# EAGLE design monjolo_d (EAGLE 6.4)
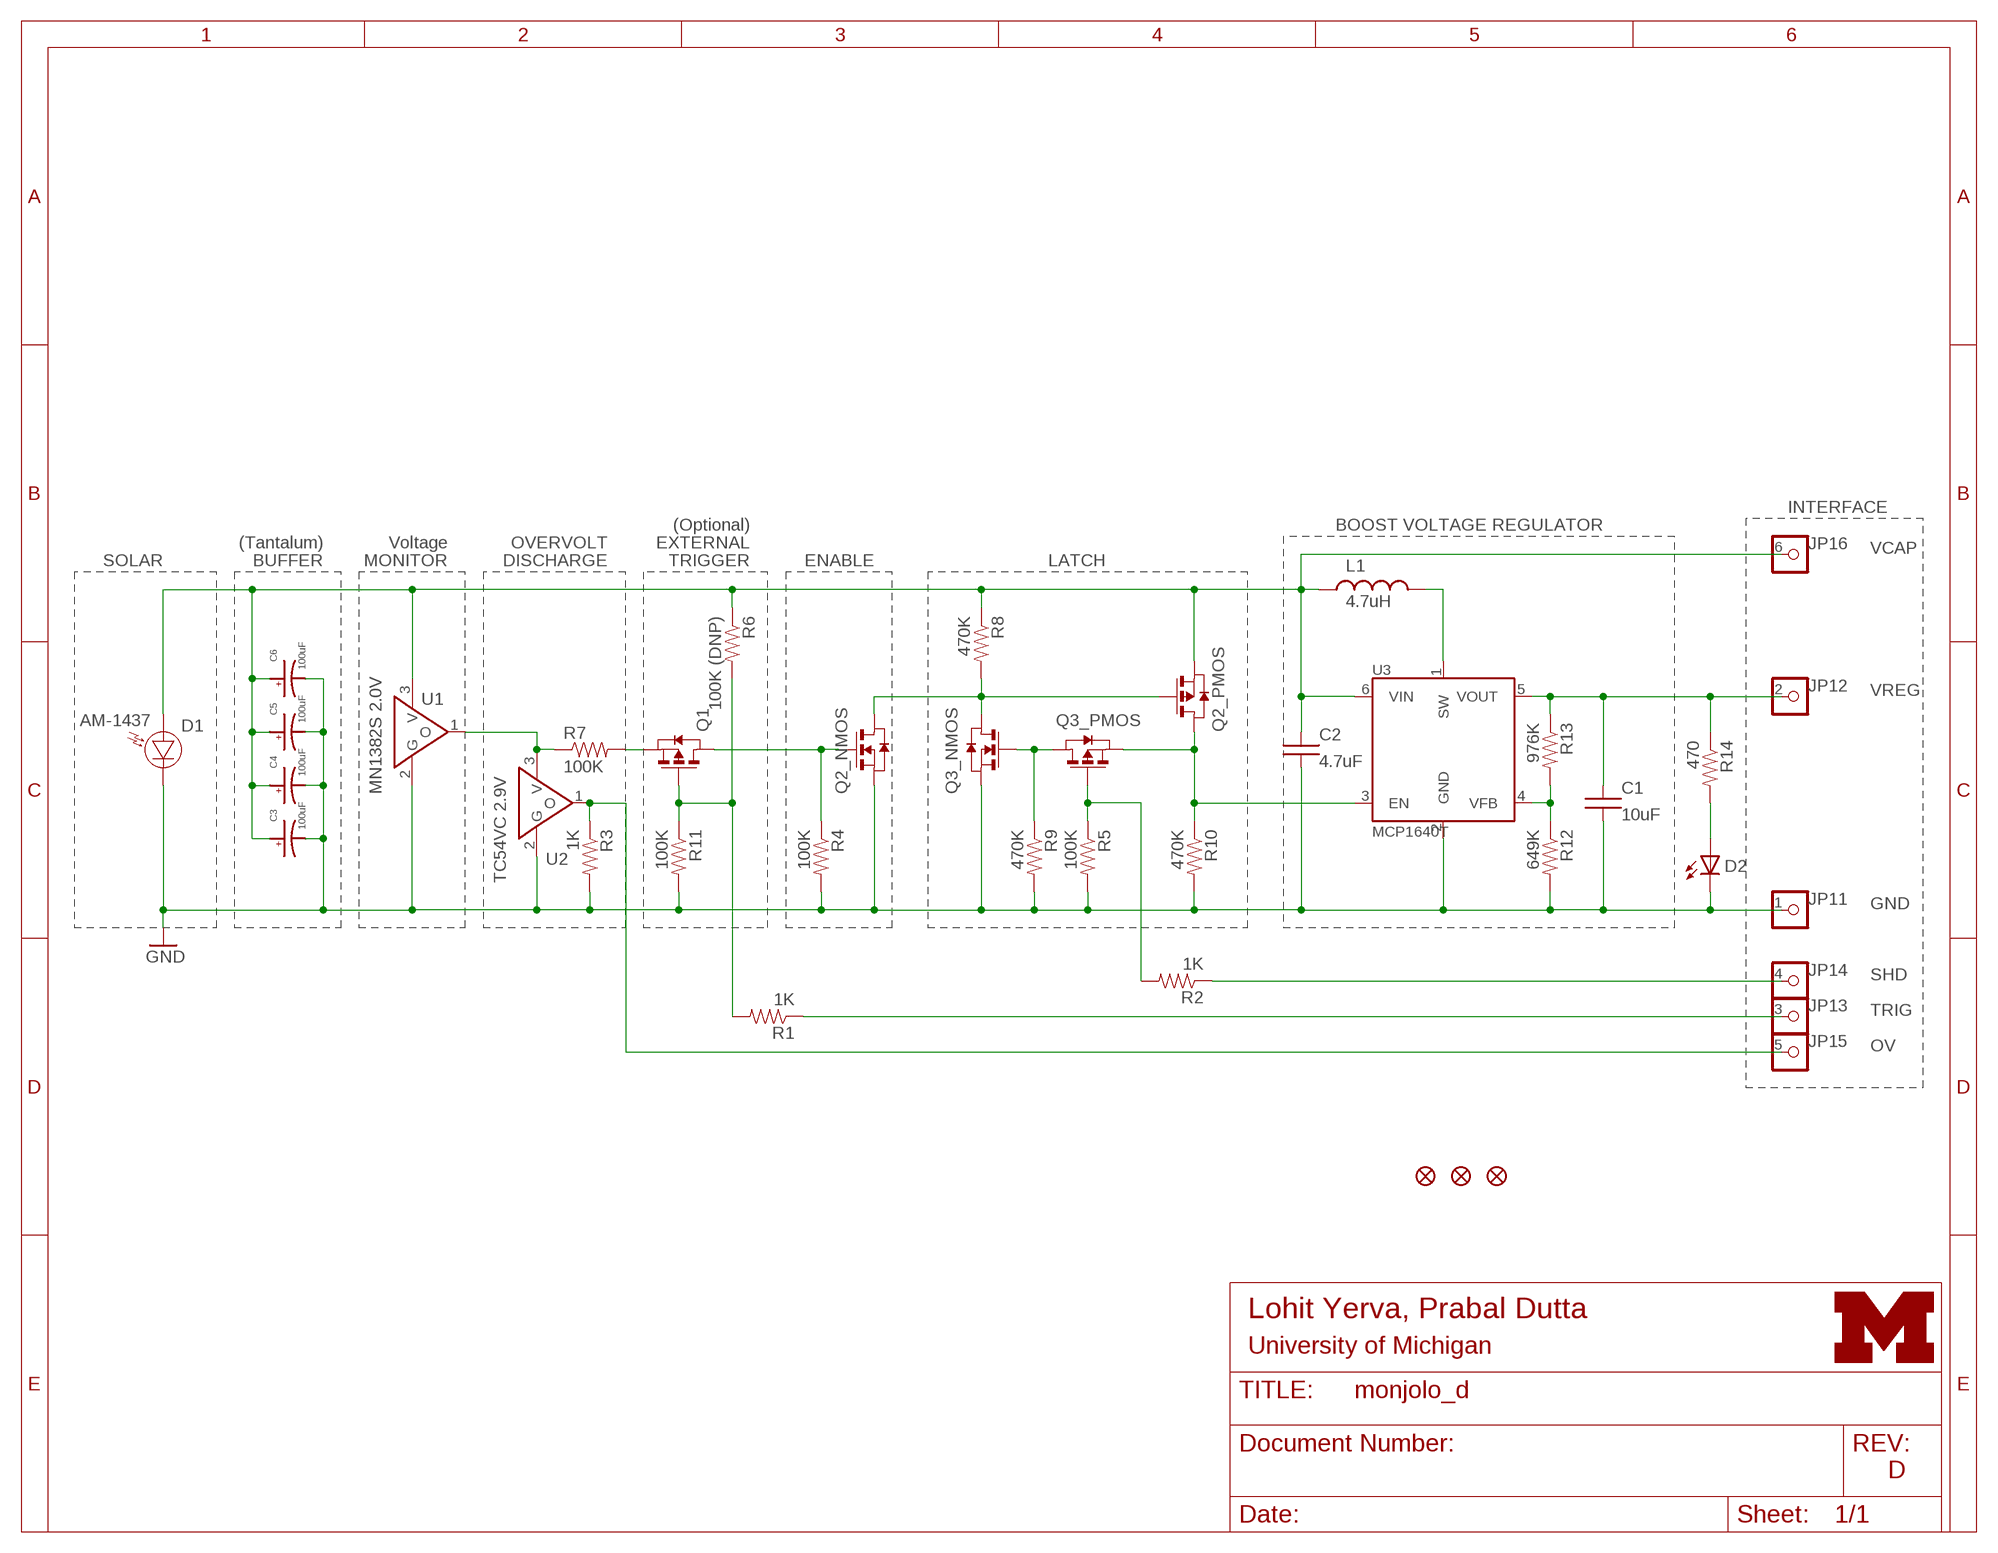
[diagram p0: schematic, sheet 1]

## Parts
C1  10uF  CAP  [R0603B]
C2  4.7uF  CAP  [R0603B]
C3  100uF  1210_CAP_POLARIZED  [CAP1210]
C4  100uF  1210_CAP_POLARIZED  [CAP1210]
C5  100uF  1210_CAP_POLARIZED  [CAP1210]
C6  100uF  1210_CAP_POLARIZED  [CAP1210]
D1  AM-1437  [AM-1437]
D2  LED0603  [LED-0603]
JP1  PINHD6  [HD6]
JP2  FIDUCIAL1X2  [FIDUCIAL-1X2]
JP3  FIDUCIAL1X2  [FIDUCIAL-1X2]
JP4  FIDUCIAL1X2  [FIDUCIAL-1X2]
L1  4.7uH  L-US  [L2828]
Q1  PMOSSOT23  [SOT-23]
Q2  DUAL_MOSFET_NP  [TSOP-6]
Q3  DUAL_MOSFET_NP  [TSOP-6]
R1  1K  RESISTOR  [R0603B]
R2  1K  RESISTOR  [R0603B]
R3  1K  RESISTOR  [R0603B]
R4  100K  RESISTOR  [R0603B]
R5  100K  RESISTOR  [R0603B]
R6  100K (DNP)  RESISTOR  [R0603B]
R7  100K  RESISTOR  [R0603B]
R8  470K  RESISTOR  [R0603B]
R9  470K  RESISTOR  [R0603B]
R10  470K  RESISTOR  [R0603B]
R11  100K  RESISTOR  [R0603B]
R12  649K  RESISTOR  [R0603B]
R13  976K  RESISTOR  [R0603B]
R14  470  RESISTOR  [R0603B]
U1  MN1382S 2.0V  MN1382S  [MINI-3DC]
U2  TC54VC 2.9V  MN1382S  [MINI-3DC]
U3  MCP1640T  MCP1640  [SOT-23-6]
U$1  UMICH_SOLID_SMALL  [UMICH_SOLID_75MIL]

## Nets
GND: C1.2 C2.2 C3.ANODE C4.ANODE C5.ANODE C6.ANODE D1.-(C) D2.C JP1.1 Q2.5(_NMOS:S) Q3.5(_NMOS:S) R3.2 R4.2 R5.2 R9.2 R10.2 R11.2 R12.2 U1.2(G) U2.2(G) U3.2(GND)
N$1: R12.1 R13.2 U3.4(VFB)
N$2: Q1.2(S) R7.2
N$3: JP1.3 R1.1
N$4: L1.2 U3.1(SW)
N$5: D2.A R14.2
N$6: Q3.1(_NMOS:G) Q3.4(_PMOS:D) R9.1
N$7: Q1.1(D) Q2.1(_NMOS:G) R4.1
N$8: JP1.4 R2.1
N$9: Q2.3(_PMOS:G) Q2.6(_NMOS:D) Q3.6(_NMOS:D) R8.2
N$12: Q3.3(_PMOS:G) R2.2 R5.1
N$13: JP1.5 R3.1 U2.1(O)
N$14: R7.1 U1.1(O) U2.3(V)
N$15: Q1.3(G) R1.2 R6.2 R11.1
N$18: Q2.4(_PMOS:D) Q3.2(_PMOS:S) R10.1 U3.3(EN)
VCAP: C2.1 C3.CATHODE C4.CATHODE C5.CATHODE C6.CATHODE D1.+(A) JP1.6 L1.1 Q2.2(_PMOS:S) R6.1 R8.1 U1.3(V) U3.6(VIN)
VREG: C1.1 JP1.2 R13.1 R14.1 U3.5(VOUT)

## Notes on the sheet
- INTERFACE
- (Optional) | BOOST VOLTAGE REGULATOR
- (Tantalum) | Voltage | OVERVOLT | EXTERNAL
- SOLAR | BUFFER | MONITOR | DISCHARGE | TRIGGER | ENABLE | LATCH | VCAP
- VREG
- GND
- SHD
- TRIG
- OV
- Lohit Yerva, Prabal Dutta
- University of Michigan
- D

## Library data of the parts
C1 C2 = Gecko:CAP
C3-C6 = Gecko:1210_CAP_POLARIZED
D1 = umich:AM-1437
D2 = umich:LED: LEDs
JP1 = Gecko:PINHD6
JP2-JP4 = SparkFun-Aesthetics:FIDUCIAL: Fiducial Alignment Points
L1 = Gecko:L-US
Q1 = berkeley-epic:PMOSSOT23: MOS FET
Q2 Q3 =  gecko_vreg_revC:DUAL_MOSFET_NP
R1-R14 = Gecko:RESISTOR
U1 U2 = umich:MN1382S
U3 = Gecko:MCP1640
U$1 = logos:UMICH_SOLID

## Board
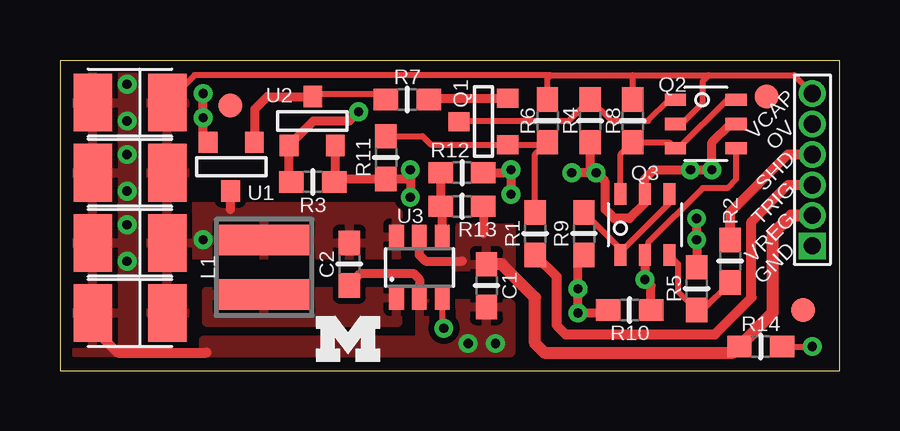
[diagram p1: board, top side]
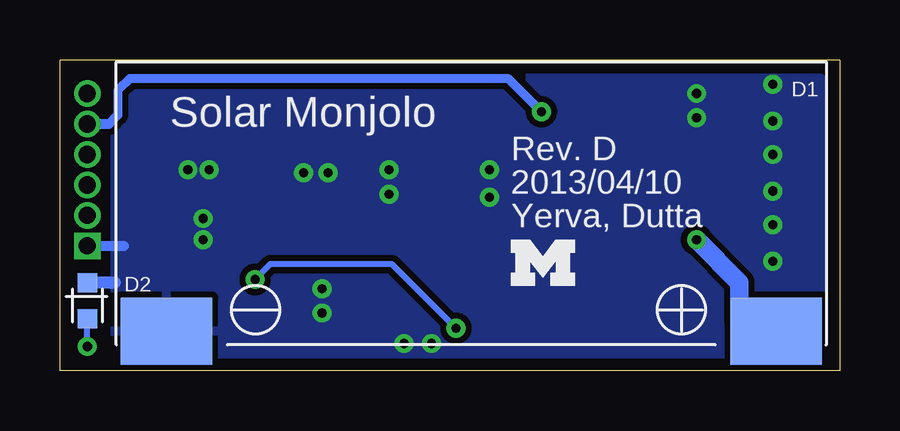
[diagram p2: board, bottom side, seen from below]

Size 32.51 x 12.95 mm. Coordinates in mm from the lower left corner, seen from the top.
Outline: 32.51,0 32.51,12.95 0,12.95 0,0 32.51,0
Copper layers (1*16): Top 0.0178mm / dielectric 59mil / Bottom 0.0178mm
Design rules "SSC-EAGLE-2Lyr_v1.0.0.3 *": minimum track width 6mil, minimum drill 14mil, track to track 6mil, track to pad 6mil, pad to pad 6mil, via to via 6mil, smd to smd 6mil, copper to edge 20mil, drill to drill 16mil, minimum pad ring 8mil, minimum via ring 8mil, stop-mask expansion 3mil, vias tented up to drill 20mil, thermal gap 10mil

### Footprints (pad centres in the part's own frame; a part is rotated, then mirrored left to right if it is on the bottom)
R0603B = smd 1.016 x 0.889: 1 -0.889,0; 2 0.889,0
CAP1210 = smd 2.4 x 1.6: ANODE 0,-1.55; CATHODE 0,1.55
AM-1437 = smd 3.81 x 2.794: + 12.7,-5.334; - -12.7,-5.334
LED-0603 = smd 0.8 x 0.8: A 0,-0.75; C 0,0.75
HD6 = drill 0.711 pad 1.016 square: 1 -2.54,0 | drill 0.711 pad 1.016: 2 -1.27,0; 3 0,0; 4 1.27,0; 5 2.54,0; 6 3.81,0
FIDUCIAL-1X2 = smd 1 x 1: 1 0,0
L2828 = smd 1.27 x 3.81: 1 -1.143,0; 2 1.143,0
SOT-23 = smd 0.787 x 0.889: 1 0.025,-1.016; 2 -0.94,1.016; 3 0.991,1.016
TSOP-6 = smd 0.508 x 0.889: 1 -1.016,-1.27; 2 0,-1.27; 3 1.016,-1.27; 4 1.016,1.27; 5 0,1.27; 6 -1.016,1.27
MINI-3DC = smd 0.787 x 0.889: 1 -0.991,-1.016; 2 0.94,-1.016; 3 0,1.016
SOT-23-6 = smd 0.61 x 1.016: 1 -0.953,-1.27; 2 0,-1.27; 3 0.953,-1.27; 4 0.953,1.27; 5 0,1.27; 6 -0.953,1.27

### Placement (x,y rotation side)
C1  17.78,3.56 270 top
C2  12.06,4.45 270 top
C3  2.92,11.18 270 top
C4  2.92,8.26 270 top
C5  2.92,5.33 270 top
C6  2.92,2.41 270 top
D1  15.37,6.99 0 bottom
D2  31.37,2.92 0 bottom
JP1  31.37,7.75 90 top
JP2  30.99,2.54 0 top
JP3  7.11,11.05 0 top
JP4  29.46,11.43 0 top
L1  8.51,4.32 270 top
Q1  17.65,10.41 270 top
Q2  26.92,10.29 270 top
Q3  24.38,6.1 0 top
R1  19.81,5.71 90 top
R2  27.94,4.57 270 top
R3  10.54,7.87 0 top
R4  22.1,10.41 270 top
R5  26.54,3.43 90 top
R6  20.32,10.41 270 top
R7  14.48,11.3 0 top
R8  23.88,10.41 270 top
R9  21.84,5.71 270 top
R10  23.75,2.54 180 top
R11  13.59,8.89 270 top
R12  16.76,8.26 0 top
R13  16.76,6.86 180 top
R14  29.21,1.02 0 top
U1  7.11,8.51 180 top
U2  10.54,10.41 0 top
U3  14.99,4.32 0 top
U$1  10.67,0.38 0 top
U$3  UMICH_SOLID_SMALL  [UMICH_SOLID_75MIL]  13.72,3.56 0 bottom

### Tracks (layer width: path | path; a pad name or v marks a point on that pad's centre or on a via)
GND  (via drill 0.38)
  Top 0.381: C2.2 12.09,3.62 12.53,4.06 14.73,4.06 14.99,3.81 U3.2 | U1.2 5.97,9.73 v5.97,10.54 v5.97,11.56 | R12.2 18.67,8.26 v18.8,8.38 v18.8,7.37 | v22.35,8.26 v21.34,8.26 | R10.2 23.11,2.41 v21.59,2.41 v21.59,3.43 21.59,4.57 R9.2 | v14.61,8.38 v14.61,7.24 14.61,8 R11.2 11.56,8 11.48,7.92 | R3.2 11.48,7.92 | 11.48,7.92 U2.2 | v26.54,6.35 v26.54,5.46 R5.2 | Q2.5 27.94,10.29 27.18,9.53 v27.18,8.38 v26.29,8.38 24.77,8.38 24.38,8 Q3.5 24.38,6.99 23.75,6.35 23.11,6.35 22.73,6.73 22.73,7.87 v22.35,8.26 | R4.2 22.1,8.51 v22.35,8.26
  Top 0.406: C6.ANODE 1.37,1.8 2.41,0.76 6.1,0.76
  Bottom 0.406: JP1.1 29.84,5.21
  Bottom 0.508: D2.C 30.36,3.67 30.23,3.68
  other vias: 18.16,1.14 17.02,1.14 2.79,4.57 2.79,6.1 2.79,7.49 2.79,9.02 2.79,10.41 2.79,11.94
  pour Bottom (isolate 0.254): 0.76,0.64 0.76,12.19 30.23,12.19 30.23,0.64
  pour Top (isolate 0.254): 5.97,1.27 5.97,0.76 18.8,0.76 18.8,2.79 14.99,2.79 14.99,1.27
  pour Top (isolate 0.305): 0.64,12.32 3.05,12.32 3.05,0.76 0.64,0.76
N$1
  Top 0.381: R12.1 R13.2 15.94,7.11 U3.4
N$2
  Top 0.381: R7.2 15.42,11.35 Q1.2
N$3
  Top 0.406: R1.1 20.7,3.94 20.7,1.91 21.08,1.52 27.3,1.52 28.83,3.05 28.83,6.22 30.35,7.75 JP1.3
N$4
  pour Top (isolate 0.254): 14.1,3.3 6.1,3.3 6.1,2.03 14.1,2.03
N$5  (via drill 0.38)
  Top 0.254: R14.2 v31.37,1.02
  Bottom 0.254: v31.37,1.02 D2.A
N$6
  Top 0.254: Q3.4 25.4,6.99 23.37,4.95 Q3.1 23.37,5.08 R9.1
N$7
  Top 0.254: Q1.1 16.66,10.41 21.21,10.41 R4.1 22.99,10.41 24.51,10.41 25.4,11.3 Q2.1
N$8
  Top 0.406: R2.1 27.94,6.6 30.35,9.02 JP1.4
N$9
  Top 0.254: Q2.6 27.81,11.3 25.78,9.27 Q2.3 25.4,9.53 R8.2 23.37,9.02 Q3.6
N$12
  Top 0.254: R2.2 26.8,2.54 R5.1 25.78,3.3 25.78,4.45 Q3.3
N$13  (via drill 0.38)
  Top 0.381: R3.1 9.55,7.98 U2.1 10.57,10.41 12.06,10.41 v12.45,10.79
  Bottom 0.381: 30.48,10.29 30.1,10.67 30.1,11.68 29.59,12.19 13.84,12.19 v12.45,10.79
  Bottom 0.406: 30.48,10.29 JP1.5
N$14
  Top 0.254: R7.1 13.34,11.56 10.79,11.56 U2.3
  Top 0.381: U2.3 8.64,11.43 8.13,10.92 8.13,9.93 U1.1
N$15
  Top 0.254: R11.1 15.11,9.78 15.47,9.42 Q1.3 20.34,9.42 R6.2 19.81,9.02 R1.2
N$18  (via drill 0.38)
  Top 0.254: U3.3 15.94,1.84 v16,1.78 | Q2.4 28.19,8 27.81,7.62 26.8,7.62 24.51,5.33 24.51,4.95 Q3.2
  Top 0.381: R10.1 24.64,3.56 v24.38,3.81 Q3.2
  Bottom 0.254: v16,1.78 18.67,4.45 23.75,4.45 v24.38,3.81
VCAP  (via drill 0.38)
  Top 0.254: 20.45,12.32 23.88,12.32 | 23.88,12.32 27.05,12.32 | 27.05,12.32 30.61,12.32 JP1.6 | Q2.2 25.91,10.29 26.8,11.18 26.8,12.06 27.05,12.32 | R6.1 20.32,12.19 20.45,12.32 | R8.1 23.88,12.32 | 20.45,12.32 5.61,12.32 C3.CATHODE
  Top 0.381: 7.11,6.73 U1.3
  Bottom 0.762: D1.+ 4.19,2.08 4.19,3.68 v5.97,5.46
  pour Top (isolate 0.254): 5.21,6.86 14.1,6.86 14.1,4.83 5.21,4.83 5.21,2.29 3.81,2.29 3.81,11.94 5.21,11.94
VREG
  Top 0.381: U3.5 14.99,4.83 15.24,4.57 16.76,4.57 | R13.1 17.65,5.71
  Top 0.508: C1.1 18.41,4.45 19.81,3.05 19.81,1.14 20.19,0.76 28.07,0.76 R14.1 29.72,2.41 29.72,5.71 30.48,6.48 JP1.2
  pour Top (isolate 0.254): 16.51,5.97 18.8,5.97 18.8,4.32 16.51,4.32

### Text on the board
tPlace: VCAP | OV | SHD | TRIG | VREG | GND
bPlace: Solar Monjolo | Rev. D | 2013/04/10 | Yerva, Dutta
tValues: VCAP | N_P_MOS | OV | PMOS | SHD | TRIG | N_P_MOS | GND | VREG

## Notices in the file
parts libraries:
SparkFun-Aesthetics: Licensing: CC v3.0 Share-Alike You are welcome to use this library for commercial purposes.
